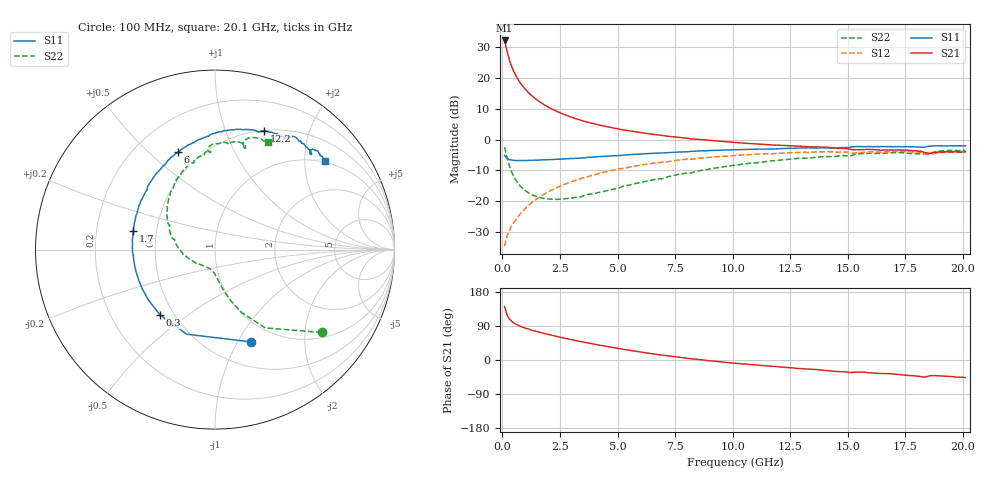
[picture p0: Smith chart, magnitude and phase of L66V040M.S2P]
!  Infineon Technologies AG
! BFR380L3 , PF131585-7, No.6, Th 09.10.01, soldered on pcb-board, measured with PP GSG850
!  Vce=6.0 V,  Ic=40.0 mA
! Common Emitter S-Parameters:  15. November 2001
#  GHz  S  MA  R  50
! f  S11  S21  S12  S22
! GHz  Mag  Ang  Mag  Ang  Mag  Ang  Mag  Ang
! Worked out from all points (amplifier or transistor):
!   201 points, 100 MHz to 20.1 GHz, reference 50 ohm
!   highest |S21| = 32.0 dB at 100 MHz (marker M1)
!   |S21| within 3 dB of that: start of sweep to 190 MHz
!   unconditionally stable (mu >= 1): 1.146 GHz to 4.301 GHz
!   at 3.4 GHz: K = 1.02, MAG = 8.6 dB, |S12| = -12.6 dB
!   at 10.1 GHz: K = 0.94, MSG = 2.1 dB, |S12| = -5.2 dB
!   at 20.1 GHz: K = 0.99, MSG = 0.1 dB, |S12| = -4.1 dB
!   S11 on the Smith chart (normalised r, x): 100 MHz: 0.77, -1.13; 300 MHz: 0.42, -0.40; 1.7 GHz: 0.37, +0.10; 6 GHz: 0.38, +0.62; 12.2 GHz: 0.50, +1.37; 20.1 GHz: 0.96, +2.52
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0.1  0.5511 -68.8  39.89 140.7  0.01889 62.0  0.7526 -37.8
0.2  0.4969 -108.5  27.18 119.9  0.02736 57.7  0.5187 -57.2
0.3  0.4755 -130.2  19.81 109.2  0.03376 57.1  0.3831 -66.9
0.4  0.4652 -143.3  15.41 102.6  0.03947 58.9  0.3029 -72.5
0.5  0.4602 -152.6  12.55 97.8  0.04533 60.9  0.2519 -76.4
0.6  0.4572 -159.6  10.57 94.2  0.0515 62.7  0.2171 -79.2
0.7  0.4564 -164.8  9.135 91.2  0.05747 63.9  0.1922 -81.7
0.8  0.4563 -169.2  8.033 88.5  0.06411 65.0  0.1737 -83.8
1  0.4567 -176.1  6.483 84.1  0.07691 66.3  0.1481 -87.8
1.2  0.4607 178.3  5.431 80.2  0.08997 66.8  0.1328 -91.7
1.4  0.4636 173.6  4.682 76.8  0.1032 66.9  0.1226 -95.5
1.7  0.4681 167.2  3.887 71.9  0.1231 66.4  0.1135 -101.6
2.4  0.4801 154.9  2.811 61.6  0.169 63.7  0.1078 -116.3
3.5  0.5034 138.6  1.996 47.4  0.24 57.6  0.1215 -137.5
4.6  0.5384 125.4  1.594 35.0  0.3072 50.7  0.1514 -159.6
6  0.582 110.6  1.297 20.9  0.3844 41.3  0.2027 178.3
6.8  0.6036 102.9  1.177 14.0  0.4254 35.6  0.2311 167.0
10.1  0.6845 78.5  0.8946 -8.4  0.5521 13.9  0.3846 131.9
12.2  0.7174 67.4  0.8039 -19.1  0.6066 0.9  0.4707 112.9
13.5  0.7306 60.9  0.762 -24.8  0.6246 -7.1  0.5097 102.9
16.8  0.7665 48.3  0.6783 -35.9  0.6337 -23.5  0.6074 80.7
20.1  0.789 38.7  0.6348 -46.2  0.627 -37.5  0.6696 63.8
